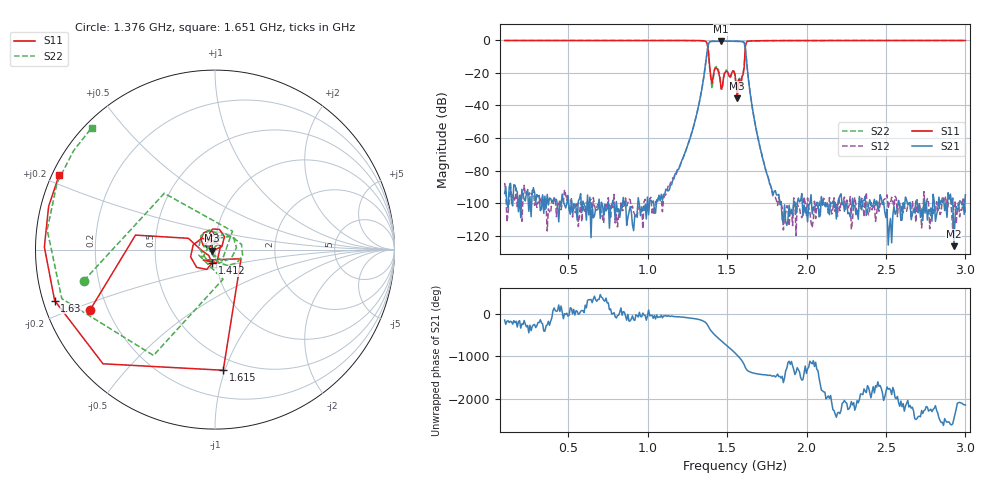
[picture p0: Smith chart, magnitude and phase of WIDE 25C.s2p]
!Agilent Technologies,E8364B,MY43040699,A.07.50.67
!Agilent E8364B: A.07.50.67
!Date: Wednesday, June 25, 2025 05:42:03
!Correction: S11(Full 2 Port(1,2))
!S21(Full 2 Port(1,2))
!S12(Full 2 Port(1,2))
!S22(Full 2 Port(1,2))
!S2P File: Measurements: S11, S21, S12, S22:
# Hz S  dB  R 50
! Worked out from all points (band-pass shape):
!   401 points, 100 MHz to 3 GHz, reference 50 ohm
!   highest |S21| = -0.46 dB at 1.463 GHz (marker M1); lowest = -126.4 dB at 2.928 GHz (marker M2)
!   |S21| within 3 dB of the highest: 1.381 GHz to 1.612 GHz (231.8 MHz wide, 15.5 % of centre)
!   lowest |S11| = -35.5 dB at 1.565 GHz (marker M3), VSWR 1.03, Z = 48.5 - j0.665 ohm
!   |S11| at or under -10 dB: 1.386 GHz to 1.612 GHz (225.8 MHz wide, 15.1 % of centre)
!   |S22| runs from -34.4 to 0.0 dB; largest |S21 - S12| = 0.00057
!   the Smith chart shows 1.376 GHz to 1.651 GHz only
!   S11 on the Smith chart (normalised r, x): 1.376 GHz: 0.14, -0.22; 1.412 GHz: 0.96, -0.15; 1.615 GHz: 0.40, -0.99; 1.63 GHz: 0.03, -0.15; 1.651 GHz: 0.02, +0.23
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1e8  -0.07 168.7  -94.10 -147.8  -87.56 159.0  -0.04 168.6
5.8575e8  -0.13 112.2  -105.55 78.9  -111.37 -78.6  -0.12 112.0
1.0715e9  -0.08 45.3  -95.12 -69.8  -96.33 -0.3  -0.09 47.7
1.20925e9  -0.07 12.7  -75.54 -74.3  -75.45 -75.1  -0.08 17.8
1.31075e9  -0.10 -36.1  -44.62 -123.8  -44.61 -123.8  -0.11 -27.4
1.376e9  -2.26 -154.3  -5.92 104.0  -5.92 104.0  -2.49 -166.7
1.41225e9  -22.27 -102.1  -0.56 -97.0  -0.56 -96.9  -23.95 80.8
1.434e9  -16.96 -163.2  -0.58 -178.2  -0.59 -178.2  -16.10 -11.3
1.463e9  -29.81 119.9  -0.46 84.2  -0.47 84.2  -29.82 -116.9
1.492e9  -18.96 124.3  -0.52 -9.1  -0.52 -9.1  -18.27 31.8
1.51375e9  -22.09 94.8  -0.49 -79.1  -0.50 -79.1  -22.06 -72.4
1.55e9  -20.97 53.8  -0.55 157.6  -0.55 157.6  -21.22 77.1
1.5645e9  -35.47 -156.0  -0.55 102.9  -0.55 102.9  -34.41 178.5
1.58625e9  -28.57 33.5  -0.66 10.1  -0.65 10.1  -27.78 164.1
1.61525e9  -3.43 -86.1  -4.90 174.5  -4.90 174.5  -3.33 -120.2
1.62975e9  -0.56 -162.4  -19.59 100.1  -19.59 100.0  -0.52 173.3
1.6515e9  -0.34 154.6  -36.65 58.4  -36.65 58.3  -0.30 135.3
1.753e9  -0.17 89.0  -82.76 -9.2  -82.36 -6.6  -0.16 76.5
2.03575e9  -0.09 33.2  -106.68 -99.7  -115.04 -18.7  -0.09 24.8
2.5215e9  -0.07 -15.4  -114.60 38.8  -99.57 -0.4  -0.07 -22.2
2.9275e9  -0.06 -47.1  -126.43 37.9  -100.09 -44.1  -0.06 -53.3
3e9  -0.06 -52.4  -94.90 11.9  -106.92 139.6  -0.06 -58.4
